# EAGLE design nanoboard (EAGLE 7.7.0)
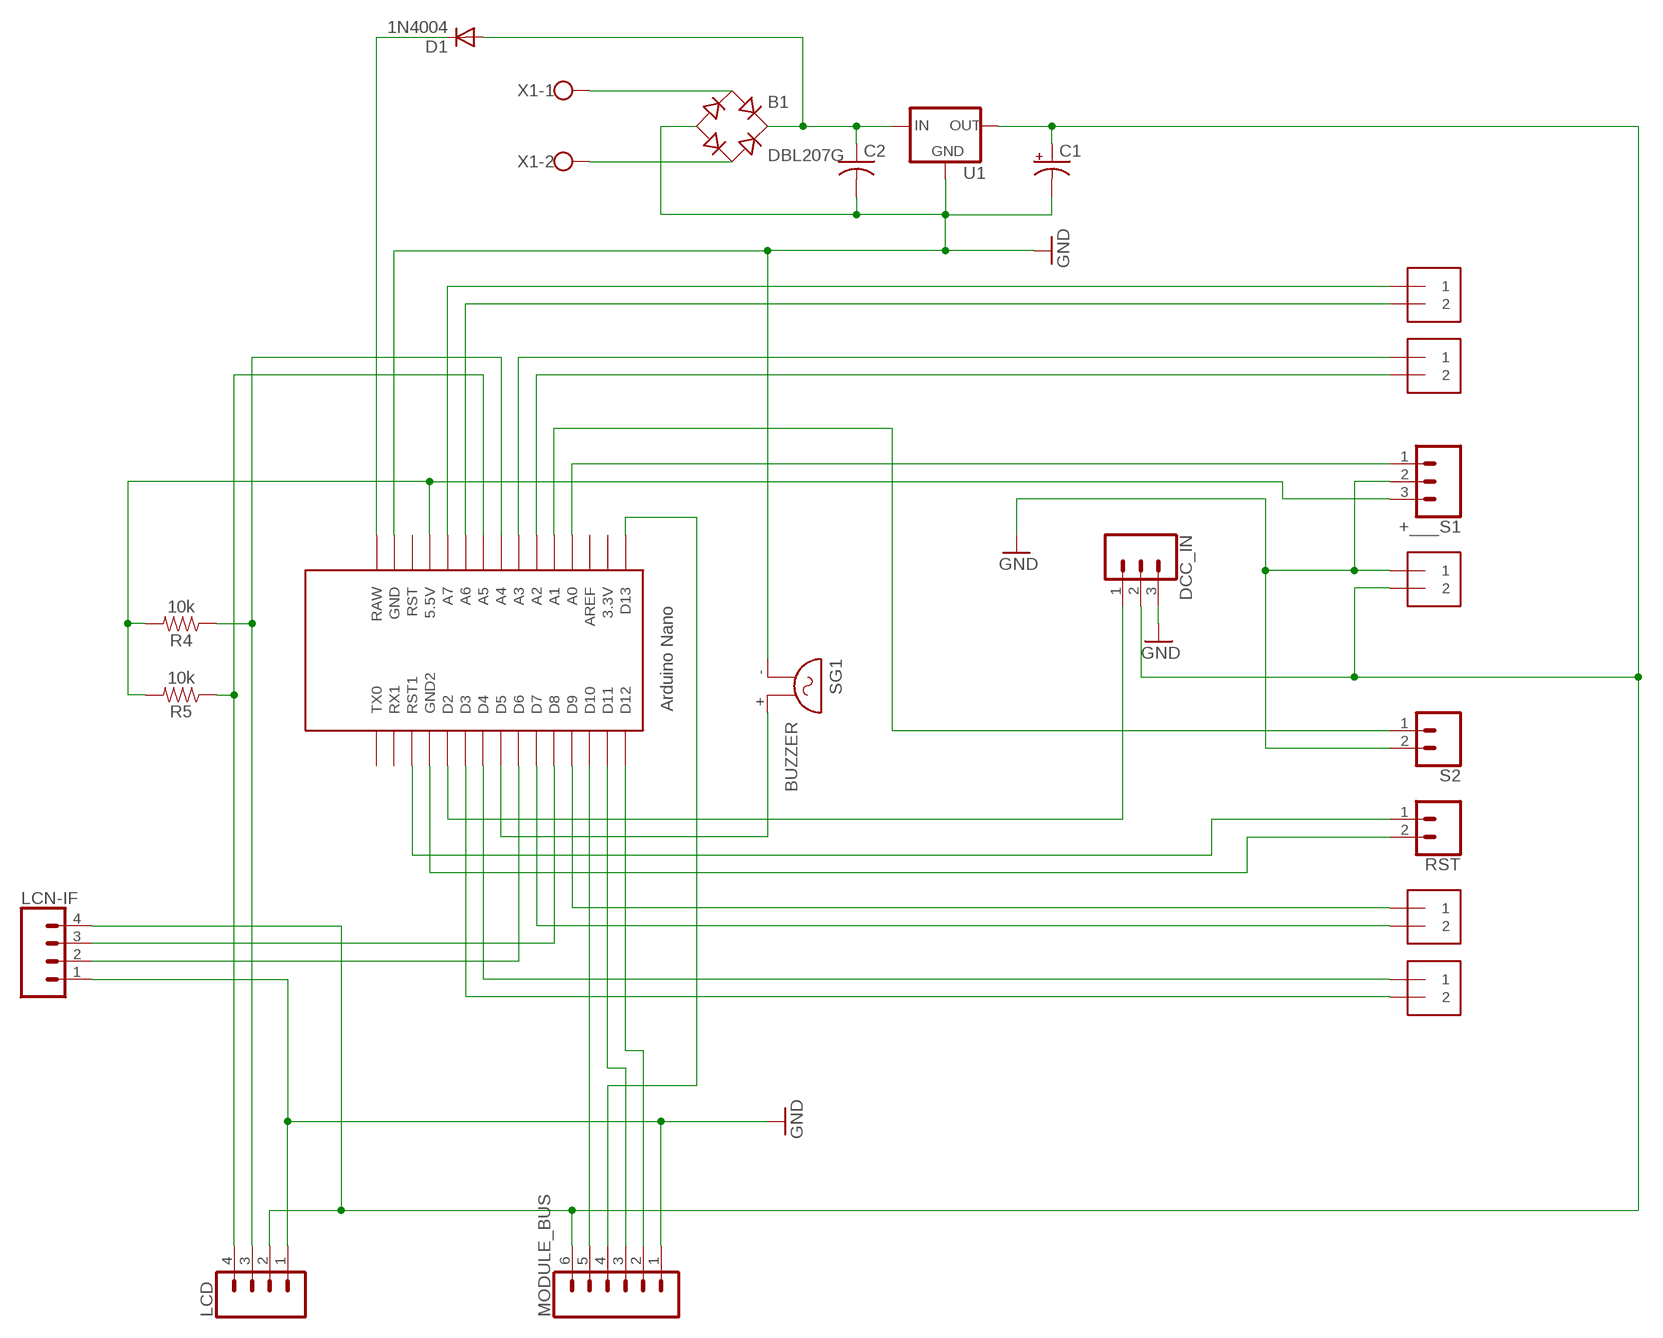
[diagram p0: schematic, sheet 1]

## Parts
+___S1  CONN_03  [1X03]
B1  DBL207G  [DB]
C1  100UF-POLAR-RADIAL-2.5MM-25V-20%  [CPOL-RADIAL-2.5MM-6.5MM]
C2  C-US025-025X050  [C025-025X050]
D1  1N4004  [DO41-10]
DCC_IN  CONN_03  [1X03]
GN_+5V  1X2-3.5MM  [1X2-3.5MM]
LCD  CONN_04  [1X04]
LCN-IF  CONN_04  [1X04]
MODULE_BUS  CONN_06SILK_FEMALE_PTH  [1X06]
P2_P1  1X2-3.5MM  [1X2-3.5MM]
P4_P3  1X2-3.5MM  [1X2-3.5MM]
P6_P5  1X2-3.5MM  [1X2-3.5MM]
P8_P7  1X2-3.5MM  [1X2-3.5MM]
R4  10k  10KOHM-HORIZ-1/4W-1%  [AXIAL-0.3]
R5  10k  10KOHM-HORIZ-1/4W-1%  [AXIAL-0.3]
RST  CONN_02  [1X02]
S2  CONN_02  [1X02]
SG1  BUZZER  [F/QMX]
U1  V_REG_78XXSINK  [TO220-IGO]
U$1  NANO_V3  [NANO]
X1  W237-102  [W237-102]

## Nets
GND: +___S1.2 B1.- C1.2(-) C2.2 DCC_IN.3 GN_+5V.1 LCD.1 LCN-IF.1 MODULE_BUS.1 S2.2 SG1.- U1.GND U$1.GND
N$1: MODULE_BUS.4 U$1.D13
N$2: LCN-IF.3 U$1.D8
N$3: LCN-IF.2 U$1.D6
N$4: P4_P3.1 U$1.D4
N$5: P4_P3.2 U$1.D3
N$6: B1.+ C2.1 D1.A U1.IN
N$7: RST.2 U$1.GND1(GND2)
N$8: C1.1(+) DCC_IN.2 GN_+5V.2 LCD.2 LCN-IF.4 MODULE_BUS.6 U1.OUT
N$9: RST.1 U$1.RST1
N$10: LCD.3 R4.P$1 U$1.A4
N$11: LCD.4 R5.P$1 U$1.A5
N$12: S2.1 U$1.A1
N$13: P8_P7.2 U$1.A6
N$14: +___S1.1 U$1.A0
N$15: P2_P1.2 U$1.A2
N$16: P2_P1.1 U$1.A3
N$17: DCC_IN.1 U$1.D2
N$18: MODULE_BUS.5 U$1.D10
N$19: MODULE_BUS.3 U$1.D11
N$20: MODULE_BUS.2 U$1.D12
N$21: D1.C U$1.RAW
N$22: P8_P7.1 U$1.A7
N$23: B1.AC2 X1.2
N$24: P6_P5.1 U$1.D9
N$25: P6_P5.2 U$1.D7
N$28: B1.AC1 X1.1
N$29: SG1.+ U$1.D5
N$31: +___S1.3 R4.P$2 R5.P$2 U$1.5V(5.5V)
Unconnected: U$1.3.3V U$1.AREF U$1.RST U$1.RX1 U$1.TX0

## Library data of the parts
+___S1 DCC_IN = plg-rms:CONN_03: Multi connection point. Often used as Generic Header-pin footprint for 0.1 inch spaced/style header connections On any of the 0.1 inch spaced packages, you can populate with these: Break Away Headers - Straight (PRT-00116) Break Away Male Headers - Right Angle (PRT-00553) Female Headers (PRT-00115)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
B1 = rectifier:DB?*G: Single Phase 1.0 AMP Glass Passivated Bridge Rectifier Taiwan Semiconductor Co.,Ltd. - TSC Source: http://www.taiwansemi.com/TSCbig5/ezcatfiles/cust/img/img/db101g.pdf http://www.ts.com.tw/db/pictures/modules/PDT/PDT060207001/DBLS201G.pdf
C1 = SparkFun-Capacitors:100UF-POLAR: 100µF polarized capacitors; PROD_ID: CAP-08439; VALUE: 100uF
C2 = adafruit:C-US: CAPACITOR, American symbol
D1 = diode:1N4004: DIODE
GN_+5V P2_P1 P4_P3 P6_P5 P8_P7 = plg-rms:1X2: 3.5mm Terminal block
LCD LCN-IF = SparkFun-Connectors:CONN_04: Multi connection point. Often used as Generic Header-pin footprint for 0.1 inch spaced/style header connections On any of the 0.1 inch spaced packages, you can populate with these: Break Away Headers - Straight (PRT-00116) Break Away Male Headers - Right Angle (PRT-00553) Female Headers (PRT-00115)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; PROD_ID: CONN-09696
MODULE_BUS = SparkFun-Connectors:CONN_06: Multi connection point. Often used as Generic Header-pin footprint for 0.1 inch spaced/style header connections On any of the 0.1 inch spaced packages, you can populate with these: Break Away Headers - Straight (PRT-00116) Break Away Male Headers - Right Angle (PRT-00553) Female Headers (PRT-00115)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; PROD_ID: CONN-08437
R4 R5 = SparkFun-Resistors:10KOHM: 10kΩ resistor; PROD_ID: RES-12183
RST S2 = SparkFun-Connectors:CONN_02: Multi connection point. Often used as Generic Header-pin footprint for 0.1 inch spaced/style header connections
SG1 = plg-rms:BUZZER: BUZZER; OC_FARNELL: unknown; OC_NEWARK: unknown
U1 = SparkFun-IC-Power:V_REG_78XX: Voltage Regulator Standard 78xx regulator. IGO (Input Ground Output). Spark Fun Electronics SKU : COM-00107
U$1 = plg-rms:NANO_V3: Arduino Nano
X1 = plg-rms:W237-102: WAGO SCREW CLAMP; MPN: 237-102; OC_FARNELL: unknown; OC_NEWARK: 70K9898

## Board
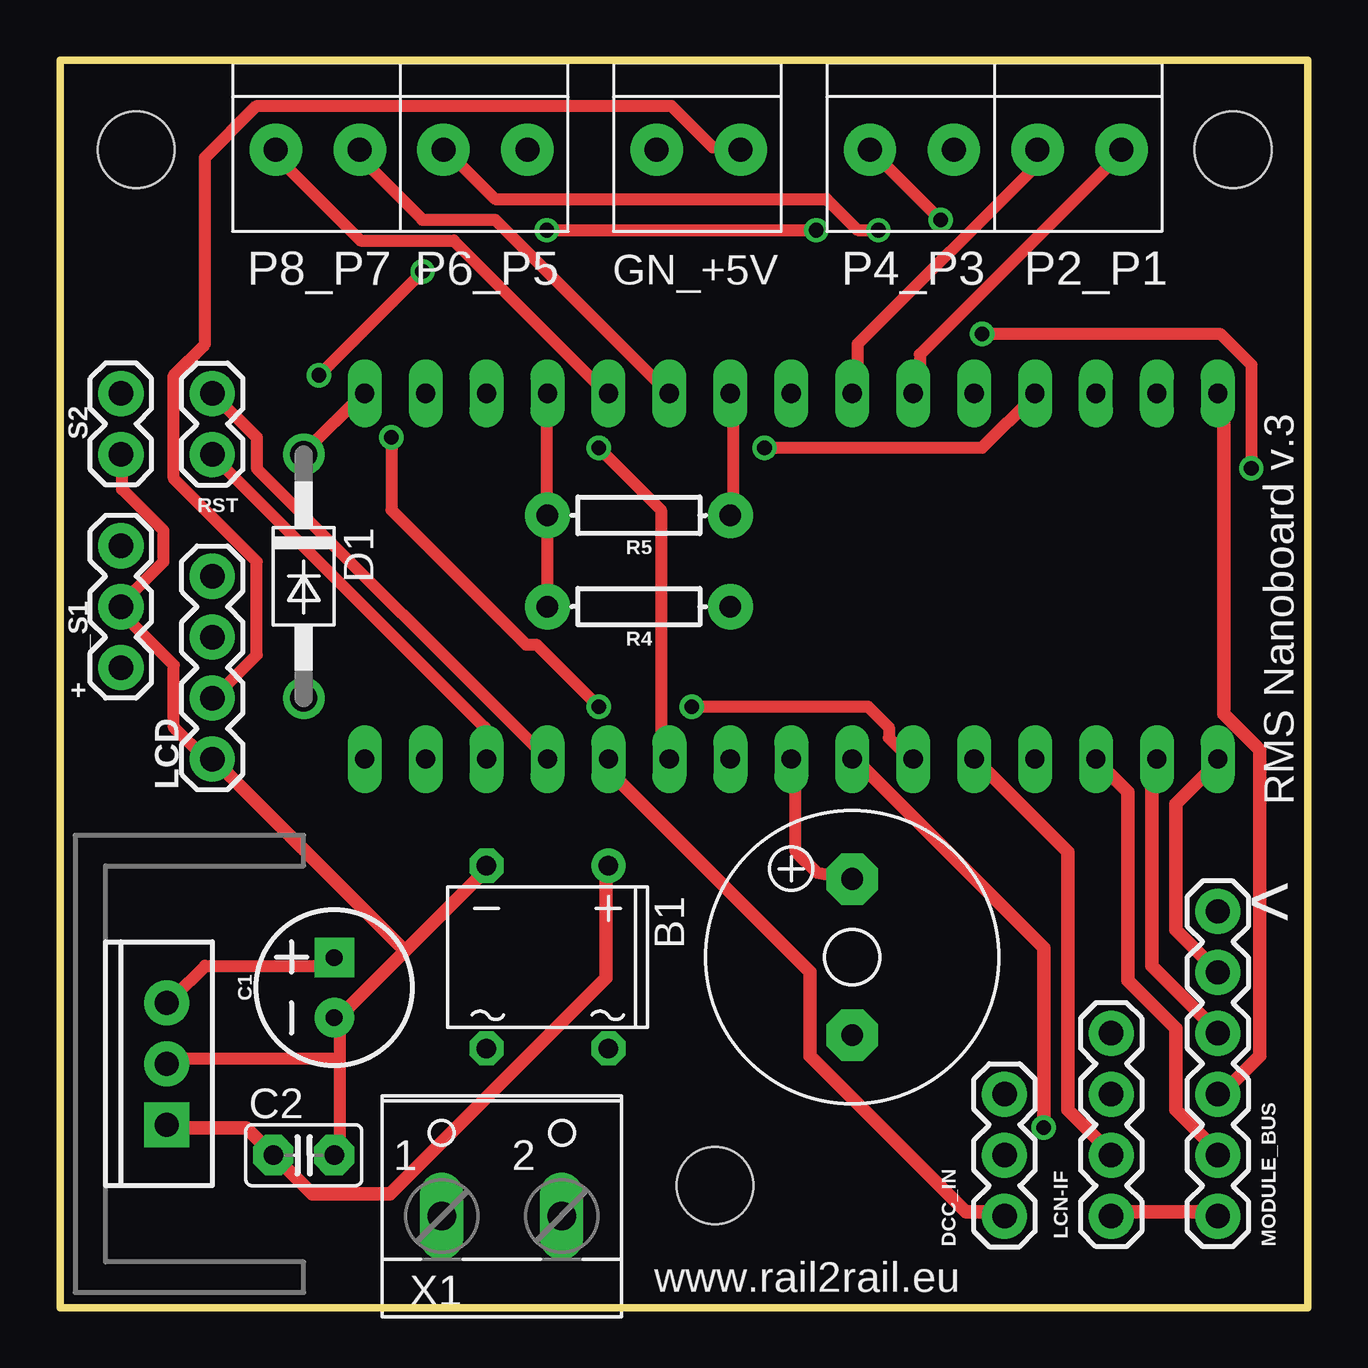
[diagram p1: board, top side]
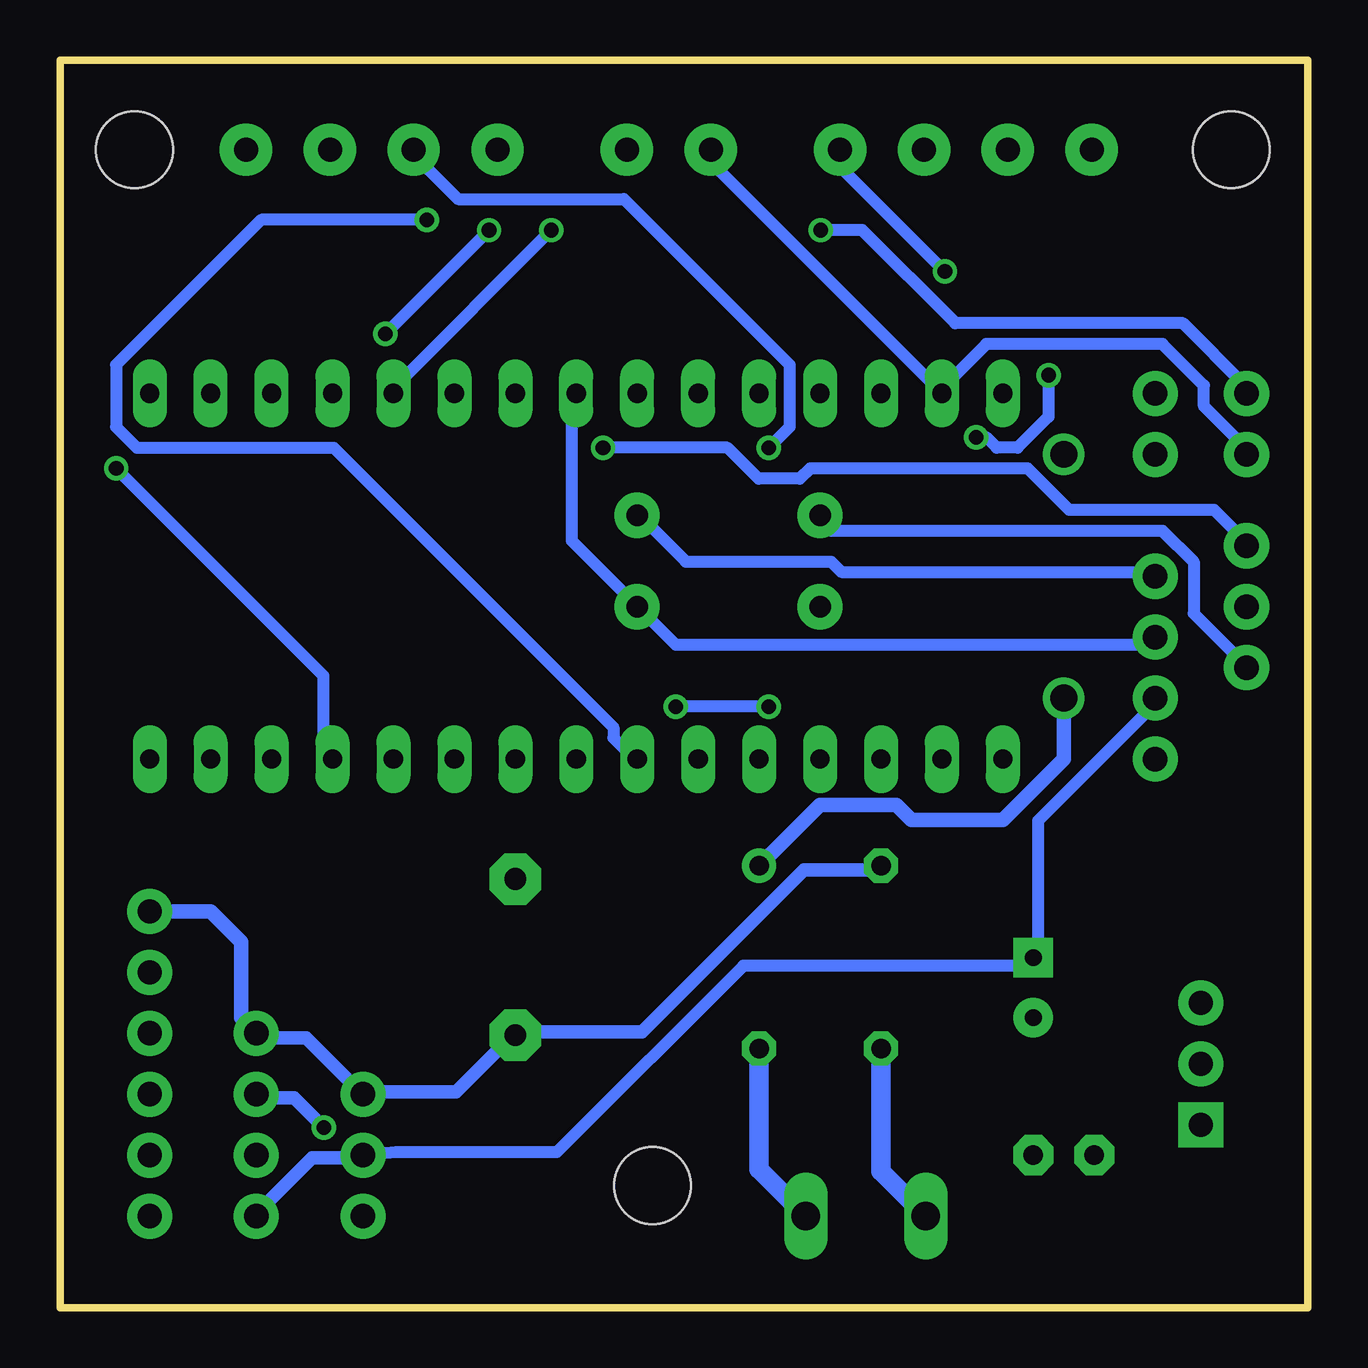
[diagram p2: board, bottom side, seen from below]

Size 52 x 52 mm. Coordinates in mm from the lower left corner, seen from the top.
Outline: 0,0 52,0 52,52 0,52 0,0
Copper layers (1*16): Top 0.035mm / dielectric 1.5mm / Bottom 0.035mm
Design rules "default *": minimum track width 22mil, minimum drill 24mil, track to track 14mil, track to pad 14mil, pad to pad 14mil, via to via 14mil, smd to smd 8mil, copper to edge 40mil, drill to drill 8mil, minimum pad ring 12mil, minimum via ring 8mil, stop-mask expansion 4mil, vias tented up to drill 0mil, thermal gap 10mil
Holes 3.2 mm at 3.17,48.26 48.9,48.26 27.3,5.08

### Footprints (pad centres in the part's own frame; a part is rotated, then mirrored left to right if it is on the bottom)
1X03 = drill 1.016 pad 1.88: 1 0,0; 2 2.54,0; 3 5.08,0
DB = drill 0.813: + -2.54,-3.81 | drill 0.813 octagon: - 2.54,-3.81; AC1 2.54,3.81; AC2 -2.54,3.81
CPOL-RADIAL-2.5MM-6.5MM = drill 0.7 pad 1.651 square: 1 1.25,0 | drill 0.7 pad 1.651: 2 -1.25,0
C025-025X050 = drill 0.813 pad 1.676 octagon: 1 -1.27,0; 2 1.27,0
DO41-10 = drill 1.118: A 5.08,0; C -5.08,0
1X2-3.5MM = drill 1 pad 2.184: 1 1.8,0; 2 -1.7,0
1X04 = drill 1.016 pad 1.88: 1 0,0; 2 2.54,0; 3 5.08,0; 4 7.62,0
1X06 = drill 1.016 pad 1.88: 1 0,0; 2 2.54,0; 3 5.08,0; 4 7.62,0; 5 10.16,0; 6 12.7,0
AXIAL-0.3 = drill 0.9 pad 1.88: P$1 -3.81,0; P$2 3.81,0
1X02 = drill 1.016 pad 1.88: 1 0,0; 2 2.54,0
F/QMX = drill 0.914 pad 2.159 octagon: + 3.251,0; - -3.251,0
TO220-IGO = drill 1 pad 1.88: GND 0,0; OUT 2.54,0 | drill 1 pad 1.88 square: IN -2.54,0
NANO = drill 0.8 long: 3.3V -10.16,24.13; 5V -10.16,-1.27; A0 -10.16,19.05; A1 -10.16,16.51; A2 -10.16,13.97; A3 -10.16,11.43; A4 -10.16,8.89; A5 -10.16,6.35; A6 -10.16,3.81; A7 -10.16,1.27; AREF -10.16,21.59; D2 5.08,1.27; D3 5.08,3.81; D4 5.08,6.35; D5 5.08,8.89; D6 5.08,11.43; D7 5.08,13.97; D8 5.08,16.51; D9 5.08,19.05; D10 5.08,21.59; D11 5.08,24.13; D12 5.08,26.67; D13 -10.16,26.67; GND -10.16,-6.35; GND1 5.08,-1.27; RAW -10.16,-8.89; RST -10.16,-3.81; RST1 5.08,-3.81; RX1 5.08,-6.35; TX0 5.08,-8.89
W237-102 = drill 1.194 long: 1 -2.5,-1.27; 2 2.5,-1.27

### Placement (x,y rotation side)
+___S1  2.54,31.75 270 top
B1  20.32,14.61 180 top
C1  11.43,13.34 90 top
C2  10.16,6.35 0 top
D1  10.16,30.48 270 top
DCC_IN  39.37,3.81 90 top
GN_+5V  26.67,48.26 180 top
LCD  6.35,22.86 90 top
LCN-IF  43.81,11.43 270 top
MODULE_BUS  48.26,16.51 270 top
P2_P1  42.55,48.26 180 top
P4_P3  35.56,48.26 180 top
P6_P5  17.78,48.26 180 top
P8_P7  10.79,48.26 180 top
R4  24.13,29.21 180 top
R5  24.13,33.02 180 top
RST  6.35,35.56 90 top
S2  2.54,38.1 270 top
SG1  33.02,14.61 90 top
U1  4.45,10.16 90 top
U$1  21.59,27.94 270 top
X1  18.41,5.08 0 top

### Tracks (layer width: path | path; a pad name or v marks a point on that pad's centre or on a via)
GND
  Top 0.508: 6.04,22.89 4.75,24.18 4.75,26.77 2.59,28.93 +___S1.2 2.59,29.36 4.32,31.09 4.32,32.38 2.59,34.11 2.59,35.41 S2.2 | 11.66,10.36 11.66,11.66 C1.2 | 11.66,10.36 11.66,6.48 C2.2 | 11.66,10.36 4.75,10.36 U1.GND
  Top 0.559: 6.04,22.89 6.25,23 LCD.1 6.5,22.75 14.38,14.88 | 14.38,14.88 11.75,12.25 11.5,12.25 C1.2 | 14.38,14.88 17.75,18.25 B1.-
  Bottom 0.508: GN_+5V.1 25.04,47.93 15.54,38.43 U$1.GND 15.11,38.43 13.39,40.16 6.04,40.16 4.32,38.43 4.32,37.57 2.59,35.84 S2.2
  Bottom 0.559: LCN-IF.1 43.75,11.5 43.75,11.25 41.75,11.25 39.5,9 DCC_IN.3 39.25,9 35.5,9 33.25,11.25 SG1.- 33,11.5 27.75,11.5 21,18.25 18,18.25 B1.-
  Bottom 0.61: LCN-IF.1 44.45,12.06 44.45,15.24 45.72,16.51 MODULE_BUS.1
N$1
  Top 0.559: U$1.D13 48.5,38 48.5,24.75 50,23.25 50,10.5 48.5,9 48.25,9 MODULE_BUS.4
N$2
  Top 0.559: U$1.D8 38.25,22.75 42,19 42,8.25 43.75,6.5 LCN-IF.3
N$3  (via drill 0.61)
  Top 0.559: v41,7.5 41,15 33.25,22.75 U$1.D6
  Bottom 0.559: v41,7.5 42.25,8.75 43.75,8.75 LCN-IF.2
N$4  (via drill 0.61)
  Top 0.508: v36.7,45.34 34.11,47.93 P4_P3.1
  Bottom 0.508: v36.7,45.34 43.61,45.34 49.66,39.29 49.66,36.7 48.79,35.84 40.59,35.84 28.93,24.18 28.93,23.75 28.07,22.89 U$1.D4
N$5  (via drill 0.61)
  Top 0.508: v22.45,35.84 25.04,33.25 25.04,22.89 U$1.D3
  Bottom 0.508: v22.45,35.84 21.59,36.7 21.59,39.29 28.5,46.2 35.41,46.2 37.13,47.93 P4_P3.2
N$6
  Top 0.559: U1.IN 4.5,7.5 7.75,7.5 8.75,6.5 C2.1 9,6.25 10.5,4.75 13.75,4.75 22.75,13.75 22.75,18.25 B1.+
  Bottom 0.61: D1.A 10.16,22.86 12.7,20.32 16.51,20.32 17.14,20.95 20.32,20.95 B1.+
N$7
  Top 0.508: U$1.GND1 8.2,34.98 8.2,36.27 6.48,38 RST.2
N$8
  Top 0.508: C1.1 11.23,14.25 6.04,14.25 4.75,12.95 U1.OUT | GN_+5V.2 28.07,48.36 27.2,48.36 25.48,50.09 8.2,50.09 6.04,47.93 6.04,40.16 4.75,38.86 4.75,34.54 8.2,31.09 8.2,27.2 6.48,25.48 LCD.2
  Top 0.559: MODULE_BUS.6 48.25,4 44,4 LCN-IF.4
  Bottom 0.508: LCD.2 6.48,25.04 11.23,20.3 11.23,14.68 C1.1 11.66,14.25 23.52,14.25 31.29,6.48 38,6.48 DCC_IN.2
  Bottom 0.559: DCC_IN.2 39.5,6.25 41.5,6.25 43.75,4 44,4 LCN-IF.4
N$9
  Top 0.508: U$1.RST1 17.7,22.89 17.7,24.18 6.48,35.41 RST.1
N$10
  Bottom 0.508: U$1.A4 30.66,38 30.66,31.95 28.07,29.36 R4.P$1 27.64,28.93 26.34,27.64 6.48,27.64 LCD.3
N$11
  Top 0.508: U$1.A5 28.07,38 28.07,33.25 R5.P$1
  Bottom 0.508: LCD.4 6.48,30.66 19.43,30.66 19.86,31.09 25.91,31.09 27.64,32.82 R5.P$1
N$12  (via drill 0.61)
  Top 0.508: v20.3,44.91 v31.52,44.91
  Bottom 0.508: v31.52,44.91 38,38.43 U$1.A1 | v20.3,44.91 18.57,44.91 14.68,41.02 5.18,41.02 2.59,38.43 S2.1
N$13
  Top 0.508: U$1.A6 25.04,38.43 18.14,45.34 15.11,45.34 12.52,47.93 P8_P7.2
N$14  (via drill 0.61)
  Top 0.508: v29.36,35.84 38.43,35.84 40.59,38 U$1.A0
  Bottom 0.508: v29.36,35.84 24.18,35.84 22.89,34.54 21.16,34.54 20.73,34.98 11.66,34.98 9.93,33.25 3.89,33.25 2.59,31.95 +___S1.1
N$15
  Top 0.508: U$1.A2 35.84,38.43 35.84,39.73 44.04,47.93 P2_P1.2
N$16
  Top 0.508: U$1.A3 33.25,38.43 33.25,40.16 41.02,47.93 P2_P1.1
N$17
  Top 0.508: 22.89,22.45 U$1.D2
  Top 0.559: U$1.D2 23,22.25 31.25,14 31.25,10.5 37.75,4 39.25,4 DCC_IN.1
N$18
  Top 0.559: U$1.D10 43.25,22.75 44.5,21.5 44.5,13.63 46.5,11.63 46.5,8.25 48.25,6.5 MODULE_BUS.5
N$19
  Top 0.559: U$1.D11 45.5,22.75 45.5,14.25 48.25,11.5 MODULE_BUS.3
N$20
  Top 0.559: U$1.D12 48.25,22.75 46.5,21 46.5,15.75 48.25,14 MODULE_BUS.2
N$21
  Top 0.508: U$1.RAW 12.52,38 10.36,35.84 D1.C
N$22
  Top 0.508: U$1.A7 22.45,38.43 16.41,44.48 12.52,44.48 9.07,47.93 P8_P7.1
N$23
  Bottom 0.813: X1.2 22.86,5.75 B1.AC2
N$24  (via drill 0.61)
  Top 0.508: v49.66,34.98 49.66,39.29 48.36,40.59 v38.43,40.59 | v34.11,44.91 33.25,44.91 31.95,46.2 18.14,46.2 16.41,47.93 P6_P5.1
  Bottom 0.508: v49.66,34.98 41.02,26.34 41.02,22.89 U$1.D9 | v34.11,44.91 v38.43,40.59
N$25  (via drill 0.61)
  Top 0.508: v26.34,25.04 33.68,25.04 34.54,24.18 34.54,23.75 35.41,22.89 U$1.D7 | v22.45,25.04 19.86,27.64 19.43,27.64 13.82,33.25 v13.82,36.27 | v15.11,43.18 v10.79,38.86
  Bottom 0.508: v22.45,25.04 v26.34,25.04 | v13.82,36.27 13.39,36.27 12.95,35.84 12.09,35.84 10.79,37.13 v10.79,38.86 | v15.11,43.18 19.86,47.93 P6_P5.2
N$28
  Bottom 0.813: X1.1 17.78,5.67 B1.AC1
N$29
  Top 0.508: U$1.D5 30.66,22.45 30.66,19 31.52,18.14 SG1.+
N$31
  Top 0.508: U$1.5V 20.3,38 20.3,33.25 R5.P$2 20.3,32.82 20.3,29.36 R4.P$2
  Bottom 0.508: +___S1.3 2.59,26.77 4.75,28.93 4.75,31.09 6.04,32.38 19.86,32.38 20.3,32.82 R5.P$2

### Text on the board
tNames: RMS Nanoboard v.3 | < | www.rail2rail.eu

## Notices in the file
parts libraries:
SparkFun-IC-Power: Licensing: Creative Commons ShareAlike 4.0 International - https://creativecommons.org/licenses/by-sa/4.0
